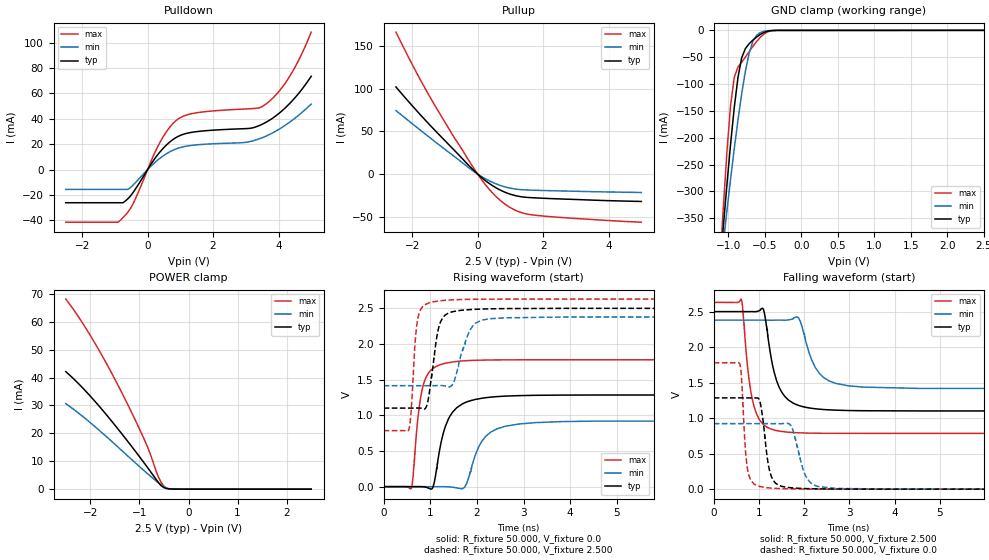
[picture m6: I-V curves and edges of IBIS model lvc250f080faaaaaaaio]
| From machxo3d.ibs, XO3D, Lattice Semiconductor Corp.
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|   Model lvc250f080faaaaaaaio
[Model] lvc250f080faaaaaaaio
Model_type I/O
Polarity   Non-Inverting
Enable   Active-Low
Vinl =  0.700V
Vinh =  1.700V
Vmeas =  1.250V
Cref =  0.0F
Rref =  1.000M
Vref =  0.0V
C_comp   4.200pF   3.800pF   7.500pF
[Temperature Range]   25.000   0.105k   -40.000
[Voltage Range]   2.500V   2.380V   2.630V
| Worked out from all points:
|   slope of the pulldown table from 0 to 0.375 V, typ, clamps not added: 27.2 ohm
|   slope of the pullup table from 0 to 0.375 V, typ, clamps not added: 32.5 ohm
|   GND clamp passes 1 mA (typ) near -0.43 V on its own axis
|   POWER clamp passes 1 mA (typ) near -0.54 V on its own axis
|   rising waveform, R_fixture 50.000, V_fixture 0.0: 20-80 % time 324ps typ, 400ps min, 193ps max; typ from 0.001 V to 1.29 V
|   rising waveform, R_fixture 50.000, V_fixture 2.500: 20-80 % time 185ps typ, 277ps min, 111ps max; typ from 1.1 V to 2.5 V
|   falling waveform, R_fixture 50.000, V_fixture 2.500: 20-80 % time 305ps typ, 376ps min, 221ps max; typ from 2.5 V to 1.1 V
|   falling waveform, R_fixture 50.000, V_fixture 0.0: 20-80 % time 158ps typ, 245ps min, 104ps max; typ from 1.29 V to 0.001 V
[Pulldown]
|Voltage   I(typ)   I(min)   I(max)
-2.5V     -26.15mA   -15.63mA   -41.49mA
-904mV    -26.15mA   -15.63mA   -41.49mA
-752mV    -26.15mA   -15.63mA   -37.84mA
-448mV    -18.28mA   -12.33mA   -27.2mA
312mV     11.8mA     7.606mA    18.2mA
768mV     23.56mA    15.16mA    36.16mA
1.376V    29.47mA    19.17mA    44.23mA
3.124V    32.48mA    22.07mA    47.96mA
3.58V     36.74mA    25.93mA    51.02mA
3.96V     43.16mA    30.94mA    59.98mA
4.34V     52.05mA    37.36mA    73.44mA
5V        73.53mA    51.63mA    108.4mA
[Pullup]
|Voltage   I(typ)   I(min)   I(max)
-2.5V     101.9mA    74.32mA    166mA
-2.068V   82.81mA    61.02mA    133mA
-1.688V   66.68mA    49.44mA    105.7mA
-700mV    27.27mA    20.17mA    41.68mA
-168mV    6.114mA    4.46mA     9.719mA
136mV     -4.568mA   -3.281mA   -7.374mA
440mV     -13.18mA   -9.386mA   -21.47mA
744mV     -19.64mA   -13.85mA   -32.38mA
1.124V    -24.85mA   -17.24mA   -41.72mA
1.58V     -27.35mA   -18.62mA   -47.12mA
2.72V     -29.25mA   -19.77mA   -51.08mA
5V        -31.92mA   -21.41mA   -56.14mA
[GND_clamp]
|Voltage   I(typ)   I(min)   I(max)
-2.5V     -2.99A     -2.35A     -4.091A
-1.123V   -455.1mA   -463.2mA   -453.7mA
-1.072V   -370.5mA   -399.5mA   -336.3mA
-1.021V   -289.2mA   -337.4mA   -228.6mA
-970mV    -212.6mA   -277.4mA   -140mA
-919mV    -143.6mA   -220.1mA   -87.39mA
-868mV    -87.38mA   -166.5mA   -68.44mA
-817mV    -50.93mA   -117.8mA   -59.12mA
-715mV    -24.98mA   -42.36mA   -39.69mA
-562mV    -7.596mA   -4.111mA   -12.93mA
-358mV    -193.4uA   -101.2uA   -309.3uA
2.5V      13.17nA    0A         -19.29uA
[POWER_clamp]
|Voltage   I(typ)   I(min)   I(max)
-2.5V     42.14mA    30.66mA    68.15mA
-2.294V   38.75mA    27.99mA    63.15mA
-2.039V   34.09mA    24.4mA     56.2mA
-1.529V   23.59mA    16.56mA    40.38mA
-1.223V   16.79mA    11.66mA    29.8mA
-917mV    9.72mA     6.817mA    18.42mA
-815mV    7.285mA    5.246mA    14.27mA
-611mV    2.32mA     2.253mA    4.314mA
-509mV    627.1uA    959.6uA    1.202mA
-458mV    269.3uA    472.4uA    476.3uA
-254mV    28.45uA    20.72uA    43.74uA
2.5V      0A         0A         0A
[Ramp]
| variable   typ   min   max
dV/dt_r   0.771/0.323n   0.553/0.395n   1.066/0.188n
dV/dt_f   0.839/0.307n   0.578/0.365n   1.106/0.221n
R_load = 50.000
[Rising Waveform]
R_fixture= 50.000
V_fixture= 0.0
V_fixture_min= 0.0
V_fixture_max= 0.0
|time   V(typ)   V(min)   V(max)
0s        1.328mV    1.004mV    1.82mV
596ps     1.372mV    1.003mV    -20.98mV
798ps     1.152mV    1.003mV    1.27V
1.038ns   -28.65mV   1.155mV    1.648V
1.278ns   748.9mV    1.03mV     1.723V
1.477ns   1.044V     -6.899mV   1.749V
1.734ns   1.175V     -8.827mV   1.765V
2.295ns   1.255V     764.8mV    1.776V
3.245ns   1.281V     898.2mV    1.779V
20ns      1.286V     923.4mV    1.779V
[Rising Waveform]
R_fixture= 50.000
V_fixture= 2.500
V_fixture_min= 2.380
V_fixture_max= 2.630
|time   V(typ)   V(min)   V(max)
0s        1.102V     1.416V     786.3mV
540ps     1.102V     1.416V     801.2mV
688ps     1.102V     1.416V     2.129V
741ps     1.103V     1.416V     2.383V
933ps     1.153V     1.416V     2.566V
1.121ns   2.019V     1.417V     2.598V
1.386ns   2.433V     1.399V     2.616V
1.85ns    2.482V     2.192V     2.627V
2.288ns   2.493V     2.355V     2.629V
20ns      2.5V       2.38V      2.63V
[Falling Waveform]
R_fixture= 50.000
V_fixture= 2.500
V_fixture_min= 2.380
V_fixture_max= 2.630
|time   V(typ)   V(min)   V(max)
0s        2.5V       2.38V      2.63V
611ps     2.5V       2.38V      2.671V
822ps     2.5V       2.38V      1.368V
1.089ns   2.542V     2.38V      916.1mV
1.299ns   1.751V     2.379V     841.6mV
1.483ns   1.39V      2.38V      814.5mV
1.87ns    1.181V     2.416V     794.7mV
2.436ns   1.122V     1.57V      787.3mV
3.308ns   1.105V     1.438V     786.4mV
20ns      1.102V     1.416V     786.1mV
[Falling Waveform]
R_fixture= 50.000
V_fixture= 0.0
V_fixture_min= 0.0
V_fixture_max= 0.0
|time   V(typ)   V(min)   V(max)
0s        1.286V     923.4mV    1.779V
577ps     1.286V     923.3mV    1.761V
757ps     1.285V     923.5mV    247.8mV
1.001ns   1.268V     923.5mV    43.03mV
1.132ns   744.8mV    923.5mV    25.35mV
1.367ns   85.32mV    923.4mV    12.27mV
1.706ns   21.41mV    897.8mV    5.085mV
2.145ns   7.163mV    88.91mV    2.513mV
2.692ns   2.829mV    12.15mV    2.01mV
20ns      1.328mV    1.004mV    1.82mV
